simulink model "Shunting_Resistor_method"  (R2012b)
settings: Solver=ode4  StartTime=0.0  StopTime=4400  FixedStep=0.001  RelTol=1e-3
undefined symbols (not defined in the file or in its folder): InitialSOC

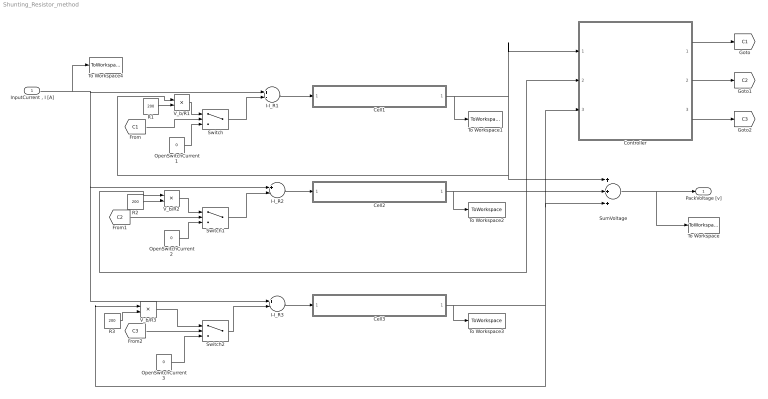
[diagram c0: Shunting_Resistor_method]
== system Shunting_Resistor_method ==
  "InputCurrent , I [A]" : Inport
  Cell1 : Subsystem
  Cell2 : Subsystem
  Cell3 : Subsystem
  Controller : Subsystem
  I-I_R1 : Sum  Inputs=+-
  I-I_R2 : Sum  Inputs=+-
  I-I_R3 : Sum  Inputs=+-
  OpenSwitchCurrent1 : Constant  Value=0
  OpenSwitchCurrent2 : Constant  Value=0
  OpenSwitchCurrent3 : Constant  Value=0
  R1 : Constant  Value=200
  R2 : Constant  Value=200
  R3 : Constant  Value=200
  SumVoltage : Sum  Inputs=+++
  Switch : Switch  Criteria=u2 > Threshold
  Switch1 : Switch  Criteria=u2 > Threshold
  Switch2 : Switch  Criteria=u2 > Threshold
  To Workspace : ToWorkspace  VariableName=PackVoltage  SampleTime=-1  SaveFormat=Structure With Time
  To Workspace1 : ToWorkspace  VariableName=CellVoltage1  SampleTime=-1  SaveFormat=Structure With Time
  To Workspace2 : ToWorkspace  VariableName=CellVoltage2  SampleTime=-1  SaveFormat=Structure With Time
  To Workspace3 : ToWorkspace  VariableName=CellVoltage3  SampleTime=-1  SaveFormat=Structure With Time
  To Workspace4 : ToWorkspace  VariableName=InputCurrent  SampleTime=-1  SaveFormat=Structure With Time
  V_b/R1 : Product  Inputs=*/
  V_b/R2 : Product  Inputs=*/
  V_b/R3 : Product  Inputs=*/
  PackVoltage [v] : Outport
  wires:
  I-I_R1/1 -> Cell1/1("InputCurrent, I_b [A]")
  Cell1/1("OutputVoltage, V_b [v]") -> To Workspace1/1, V_b/R1/1, SumVoltage/1, Controller/1(V_b1 [v])
  R1/1 -> V_b/R1/2
  I-I_R2/1 -> Cell2/1("InputCurrent, I_b [A]")
  "InputCurrent , I [A]"/1 -> To Workspace4/1, I-I_R3/1, I-I_R2/1, I-I_R1/1
  I-I_R3/1 -> Cell3/1("InputCurrent, I_b [A]")
  Switch2/1 -> I-I_R3/2
  SumVoltage/1 -> PackVoltage [v]/1, To Workspace/1
  Controller/1(Switch1_condition) -> [C1]
  Controller/2(Switch2_condition) -> [C2]
  Controller/3(Switch3_condition) -> [C3]
  [C1] -> Switch/2
  Switch/1 -> I-I_R1/2
  R2/1 -> V_b/R2/2
  Cell2/1("OutputVoltage, V_b [v]") -> To Workspace2/1, V_b/R2/1, Controller/2(V_b2 [v]), SumVoltage/2
  Switch1/1 -> I-I_R2/2
  Cell3/1("OutputVoltage, V_b [v]") -> To Workspace3/1, Controller/3(V_b3 [v]), SumVoltage/3, V_b/R3/1
  R3/1 -> V_b/R3/2
  [C3] -> Switch2/2
  [C2] -> Switch1/2
  OpenSwitchCurrent3/1 -> Switch2/3
  V_b/R3/1 -> Switch2/1
  V_b/R2/1 -> Switch1/1
  OpenSwitchCurrent2/1 -> Switch1/3
  OpenSwitchCurrent1/1 -> Switch/3
  V_b/R1/1 -> Switch/1

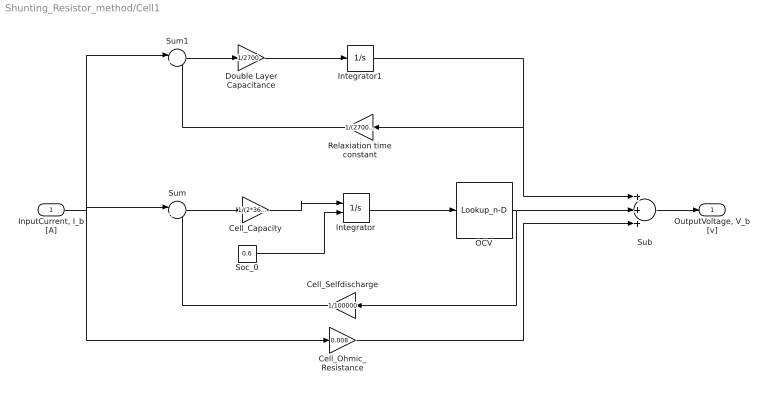
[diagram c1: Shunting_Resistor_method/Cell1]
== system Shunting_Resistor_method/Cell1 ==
  "InputCurrent, I_b [A]" : Inport
  Cell_Capacity : Gain  Gain=1/(2*3600)
  Cell_Ohmic_Resistance : Gain  Gain=0.008
  Cell_Selfdischarge : Gain  Gain=1/100000
  Double Layer Capacitance : Gain  Gain=1/2700
  Integrator : Integrator  InitialConditionSource=external  InitialCondition=InitialSOC
  Integrator1 : Integrator
  OCV : Lookup_n-D  NumberOfTableDimensions=1  BreakpointsForDimension1=[0 0.1 0.2 0.3 0.4 0.5 0.6 0.7 0.8 0.9 1]  Table=[2.25 3.2 3.25 3.25 3.3 3.3 3.3 3.35 3.35 3.35 3.75]  RndMeth=Simplest
  Relaxiation time constant : Gain  Gain=1/(2700*0.011)
  Soc_0 : Constant  Value=0.6
  Sub : Sum  Inputs=+++
  Sum : Sum  Inputs=|+-
  Sum1 : Sum  Inputs=|+-
  "OutputVoltage, V_b [v]" : Outport
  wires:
  Integrator/1 -> OCV/1
  OCV/1 -> Cell_Selfdischarge/1, Sub/2
  "InputCurrent, I_b [A]"/1 -> Sum1/1, Cell_Ohmic_Resistance/1, Sum/1
  Cell_Capacity/1 -> Integrator/1
  Cell_Selfdischarge/1 -> Sum/2
  Integrator1/1 -> Relaxiation time constant/1, Sub/1
  Relaxiation time constant/1 -> Sum1/2
  Cell_Ohmic_Resistance/1 -> Sub/3
  Sub/1 -> "OutputVoltage, V_b [v]"/1
  Sum/1 -> Cell_Capacity/1
  Double Layer Capacitance/1 -> Integrator1/1
  Sum1/1 -> Double Layer Capacitance/1
  Soc_0/1 -> Integrator/2

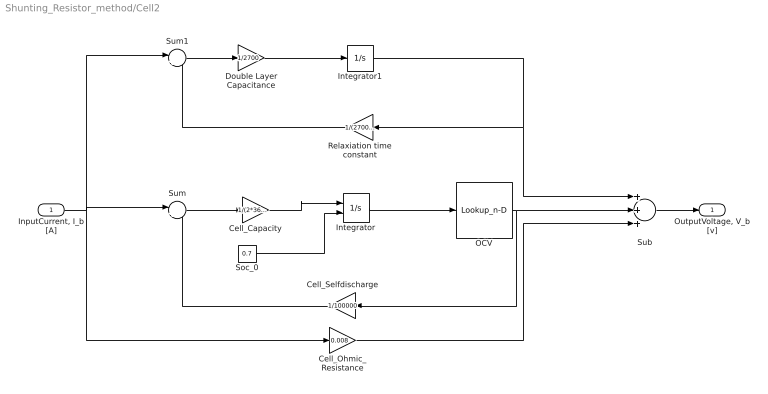
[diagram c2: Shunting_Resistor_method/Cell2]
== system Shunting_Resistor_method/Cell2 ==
  "InputCurrent, I_b [A]" : Inport
  Cell_Capacity : Gain  Gain=1/(2*3600)
  Cell_Ohmic_Resistance : Gain  Gain=0.008
  Cell_Selfdischarge : Gain  Gain=1/100000
  Double Layer Capacitance : Gain  Gain=1/2700
  Integrator : Integrator  InitialConditionSource=external  InitialCondition=InitialSOC
  Integrator1 : Integrator
  OCV : Lookup_n-D  NumberOfTableDimensions=1  BreakpointsForDimension1=[0 0.1 0.2 0.3 0.4 0.5 0.6 0.7 0.8 0.9 1]  Table=[2.25 3.2 3.25 3.25 3.3 3.3 3.3 3.35 3.35 3.35 3.75]  RndMeth=Simplest
  Relaxiation time constant : Gain  Gain=1/(2700*0.011)
  Soc_0 : Constant  Value=0.7
  Sub : Sum  Inputs=+++
  Sum : Sum  Inputs=|+-
  Sum1 : Sum  Inputs=|+-
  "OutputVoltage, V_b [v]" : Outport
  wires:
  Integrator/1 -> OCV/1
  OCV/1 -> Cell_Selfdischarge/1, Sub/2
  "InputCurrent, I_b [A]"/1 -> Sum1/1, Cell_Ohmic_Resistance/1, Sum/1
  Cell_Capacity/1 -> Integrator/1
  Cell_Selfdischarge/1 -> Sum/2
  Integrator1/1 -> Relaxiation time constant/1, Sub/1
  Relaxiation time constant/1 -> Sum1/2
  Cell_Ohmic_Resistance/1 -> Sub/3
  Sub/1 -> "OutputVoltage, V_b [v]"/1
  Sum/1 -> Cell_Capacity/1
  Double Layer Capacitance/1 -> Integrator1/1
  Sum1/1 -> Double Layer Capacitance/1
  Soc_0/1 -> Integrator/2

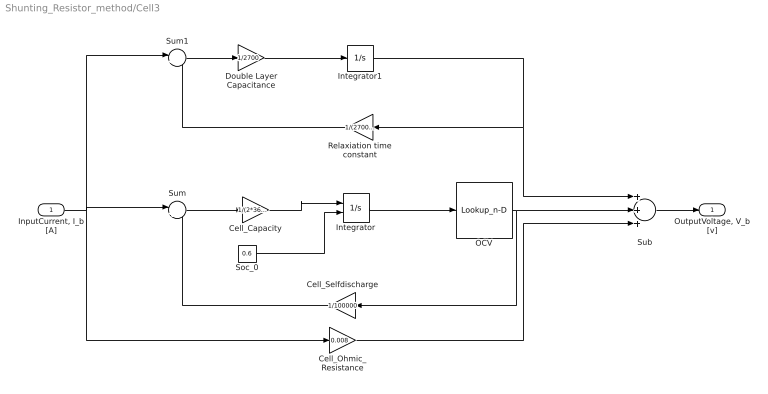
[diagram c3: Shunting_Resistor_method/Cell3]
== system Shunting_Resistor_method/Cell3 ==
  "InputCurrent, I_b [A]" : Inport
  Cell_Capacity : Gain  Gain=1/(2*3600)
  Cell_Ohmic_Resistance : Gain  Gain=0.008
  Cell_Selfdischarge : Gain  Gain=1/100000
  Double Layer Capacitance : Gain  Gain=1/2700
  Integrator : Integrator  InitialConditionSource=external  InitialCondition=InitialSOC
  Integrator1 : Integrator
  OCV : Lookup_n-D  NumberOfTableDimensions=1  BreakpointsForDimension1=[0 0.1 0.2 0.3 0.4 0.5 0.6 0.7 0.8 0.9 1]  Table=[2.25 3.2 3.25 3.25 3.3 3.3 3.3 3.35 3.35 3.35 3.75]  RndMeth=Simplest
  Relaxiation time constant : Gain  Gain=1/(2700*0.011)
  Soc_0 : Constant  Value=0.6
  Sub : Sum  Inputs=+++
  Sum : Sum  Inputs=|+-
  Sum1 : Sum  Inputs=|+-
  "OutputVoltage, V_b [v]" : Outport
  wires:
  Integrator/1 -> OCV/1
  OCV/1 -> Cell_Selfdischarge/1, Sub/2
  "InputCurrent, I_b [A]"/1 -> Sum1/1, Cell_Ohmic_Resistance/1, Sum/1
  Cell_Capacity/1 -> Integrator/1
  Cell_Selfdischarge/1 -> Sum/2
  Integrator1/1 -> Relaxiation time constant/1, Sub/1
  Relaxiation time constant/1 -> Sum1/2
  Cell_Ohmic_Resistance/1 -> Sub/3
  Sub/1 -> "OutputVoltage, V_b [v]"/1
  Sum/1 -> Cell_Capacity/1
  Double Layer Capacitance/1 -> Integrator1/1
  Sum1/1 -> Double Layer Capacitance/1
  Soc_0/1 -> Integrator/2

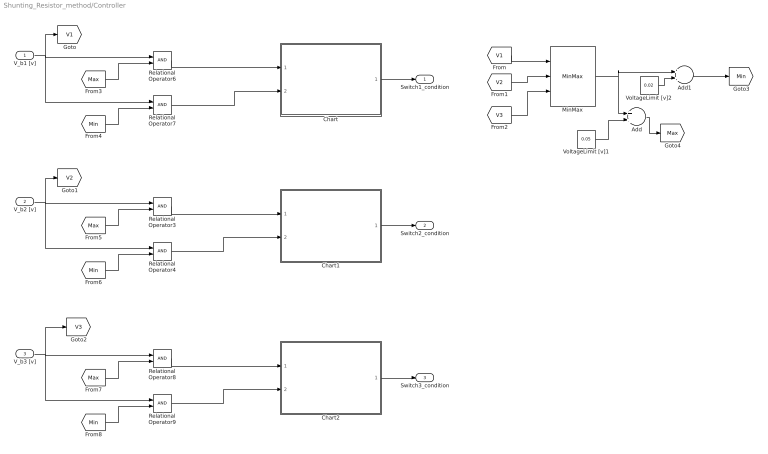
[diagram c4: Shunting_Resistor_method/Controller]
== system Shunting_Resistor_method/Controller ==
  V_b1 [v] : Inport
  V_b2 [v] : Inport  Port=2
  V_b3 [v] : Inport  Port=3
  Add : Sum
  Add1 : Sum
  Chart : Stateflow chart  TreatAsAtomicUnit=on
  Chart1 : Stateflow chart  TreatAsAtomicUnit=on
  Chart2 : Stateflow chart  TreatAsAtomicUnit=on
  MinMax : MinMax  Inputs=3
  Relational Operator{3..4,6..9} (6 alike) : RelationalOperator  OutDataTypeStr=boolean
  VoltageLimit [v]1 : Constant  Value=0.05
  VoltageLimit [v]2 : Constant  Value=0.02
  Switch1_condition : Outport
  Switch2_condition : Outport  Port=2
  Switch3_condition : Outport  Port=3
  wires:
  [Max] -> Relational Operator6/2
  Relational Operator6/1 -> Chart/1(VH)
  Chart/1(switchA) -> Switch1_condition/1
  V_b1 [v]/1 -> [V1], Relational Operator7/1, Relational Operator6/1
  [Min] -> Relational Operator7/2
  Relational Operator7/1 -> Chart/2(VL)
  [Max] -> Relational Operator3/2
  Relational Operator3/1 -> Chart1/1(VH)
  Chart1/1(switchB) -> Switch2_condition/1
  V_b2 [v]/1 -> [V2], Relational Operator4/1, Relational Operator3/1
  [Min] -> Relational Operator4/2
  Relational Operator4/1 -> Chart1/2(VL)
  [Max] -> Relational Operator8/2
  Relational Operator8/1 -> Chart2/1(VH)
  Chart2/1(switchC) -> Switch3_condition/1
  V_b3 [v]/1 -> [V3], Relational Operator9/1, Relational Operator8/1
  [Min] -> Relational Operator9/2
  Relational Operator9/1 -> Chart2/2(VL)
  [V1] -> MinMax/1
  [V2] -> MinMax/2
  [V3] -> MinMax/3
  MinMax/1 -> Add1/1, Add/1
  VoltageLimit [v]1/1 -> Add/2
  Add/1 -> [Max]
  Add1/1 -> [Min]
  VoltageLimit [v]2/1 -> Add1/2
